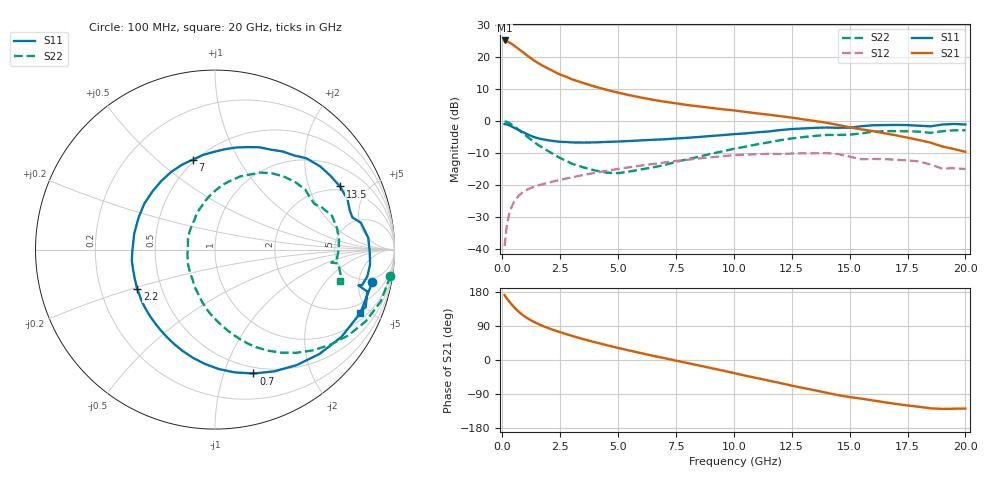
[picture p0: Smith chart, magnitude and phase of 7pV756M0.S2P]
! Infineon Technologies  Discrete & RF Semiconductors
! bfp620
! VCE = 0.75 V,  IC =  6.0 mA
! Common Emitter S-Parameters:  Sep 2002
# GHz  S  MA  R  50
!  f  S11  S21  S12  S22
! GHz  MAG  ANG  MAG  ANG  MAG  ANG  MAG  ANG
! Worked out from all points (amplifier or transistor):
!   59 points, 100 MHz to 20 GHz, reference 50 ohm
!   highest |S21| = 25.2 dB at 100 MHz (marker M1)
!   |S21| within 3 dB of that: start of sweep to 767.2 MHz
!   unconditionally stable (mu >= 1): 4.666 GHz to 11.17 GHz; 16.84 GHz to end of sweep
!   at 1 GHz: K = 0.37, MSG = 21.4 dB, |S12| = -21.8 dB
!   at 5.5 GHz: K = 1.04, MAG = 10.0 dB, |S12| = -14.5 dB
!   at 20 GHz: K = 1.55, MAG = -1.7 dB, |S12| = -15.0 dB
!   S11 on the Smith chart (normalised r, x): 100 MHz: 4.12, -7.53; 700 MHz: 0.44, -1.26; 2.2 GHz: 0.36, -0.21; 7 GHz: 0.48, +0.66; 13.5 GHz: 1.81, +3.26; 20 GHz: 1.40, -4.36
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0.1  0.8951 -11.7  18.3 171.0  0.0109 82.2  0.9886 -8.5
0.2  0.8834 -23.6  17.8 162.2  0.0239 77.8  0.9676 -17.4
0.3  0.8563 -34.6  17.05 154.3  0.035 72.1  0.9299 -25.5
0.4  0.8227 -45.0  16.19 146.9  0.0447 66.8  0.883 -32.8
0.5  0.7879 -54.8  15.29 140.0  0.0531 62.0  0.8324 -39.6
0.6  0.7543 -64.1  14.39 133.7  0.0605 57.8  0.7813 -46.0
0.7  0.7226 -72.8  13.52 127.9  0.0668 54.1  0.7316 -51.8
0.8  0.6929 -80.9  12.68 122.6  0.0723 50.9  0.6842 -57.1
1  0.6386 -95.3  11.15 113.6  0.0811 45.7  0.5975 -66.3
1.1  0.6142 -101.8  10.46 109.7  0.0847 43.7  0.5586 -70.3
1.3  0.5726 -113.6  9.262 102.8  0.0909 40.3  0.4902 -77.3
1.7  0.52 -133.3  7.518 91.3  0.1012 35.7  0.3889 -89.6
2.2  0.4854 -153.2  6.046 79.4  0.1128 31.8  0.3031 -103.3
3  0.4609 -178.8  4.508 63.8  0.1307 26.7  0.2139 -124.8
3.5  0.4588 168.9  3.939 55.0  0.1425 23.7  0.1875 -138.3
5  0.476 137.0  2.781 31.8  0.1772 13.7  0.152 173.0
7  0.5162 104.0  2.008 5.0  0.2238 -1.7  0.2031 123.9
8.5  0.5617 84.5  1.691 -14.5  0.2585 -15.2  0.2757 101.5
10.5  0.6386 60.6  1.388 -41.4  0.297 -36.8  0.3954 76.9
13.5  0.7799 26.8  0.998 -80.0  0.311 -68.6  0.5835 40.4
17  0.8681 -5.4  0.596 -115.9  0.2468 -98.9  0.6925 4.5
20  0.8797 -23.6  0.329 -128.0  0.177 -112.5  0.7168 -14.2
